(* Logix 5000 Routine export R00_CSV_Control; software revision 36.00 *)

VAR_GLOBAL   (* controller tags *)
   Create_New_CSV_File : BOOL;
   Create_New_CSV_Folder : BOOL;
   CSV_Capture_Rate_Seconds : REAL := 2.0;
   CSV_Data_Logging : BOOL := 1;
   CSV_File_Delay : TIMER := (PRE := 4000);
   CSV_Line_Count_Aux : DINT := 24844;
   CSV_Line_Count_Check_Timer : TIMER := (PRE := 5000);
   CSV_Trigger_2_Pulse : TIMER := (PRE := 1000);
   CSV_Trigger_3_Pulse : TIMER := (PRE := 1000);
   CSV_Update_Pulse : BOOL;
   CSV_Watchdog_Check_Timer : TIMER := (PRE := 5000);
   CurrentWallClock : DINT[7] := ([0] := 2025, [1] := 1, [2] := 19, [3] := 13, [4] := 49, [5] := 30, [6] := 638639);
   Data_Logger_Running : BOOL := 1;
   First_Day_Of_Calendar_Month : BOOL;
   Heartbeat_Off_Time : TIMER := (PRE := 1000);
   Heartbeat_On_Time : TIMER := (PRE := 1000);
   Line_Count : DINT := 50;
   Off_Time : TIMER := (PRE := 5000);
   On_Time : TIMER := (PRE := 100);
   ons_11 : BOOL;
   ONS_4 : BOOL;
   ONS_5 : BOOL;
   ONS_6 : BOOL;
   ONS_7 : BOOL;
   ONS_8 : BOOL := 1;
   ONS_9 : BOOL;
   Pulse_off_Time : TIMER := (PRE := 1700);
   Pulse_On_Time : TIMER := (PRE := 300);
   pulse_time_max : DINT := 3363482;
   SINKRO_File_Name : STRING := 'Report 005 Data';
   SINKRO_Folder_Name : STRING := 'Folder 003';
   SINKRO_Heartbeat : BOOL;
   SINKRO_Line_Count : DINT := 24845;
   SINKRO_New_File : BOOL;
   SINKRO_New_Folder : BOOL;
   SINKRO_Read : BOOL;
   SINKRO_Watchdog : DINT := 92;
   Start_Of_Each_Day : BOOL;
   Temp_Off : BOOL;
   Temp_Off_Time : TIMER := (PRE := 1900);
   Temp_On_Time : TIMER := (PRE := 100);
   Timer_Off_Preset_Aux : DINT := 2000;
   Trigger_1_Temp_Off : BOOL;
   Trigger_1_Timeout : TIMER := (PRE := 2000);
   Watchdog : DINT := 99;
   Watchdog_Check_Pulse : BOOL;
   Watchdog_Max : DINT := 99;
END_VAR

PROGRAM MainProgram
VAR
   CSV_Watchdog_AUx : DINT := 90;
END_VAR

ROUTINE R00_CSV_Control   (* ladder *)
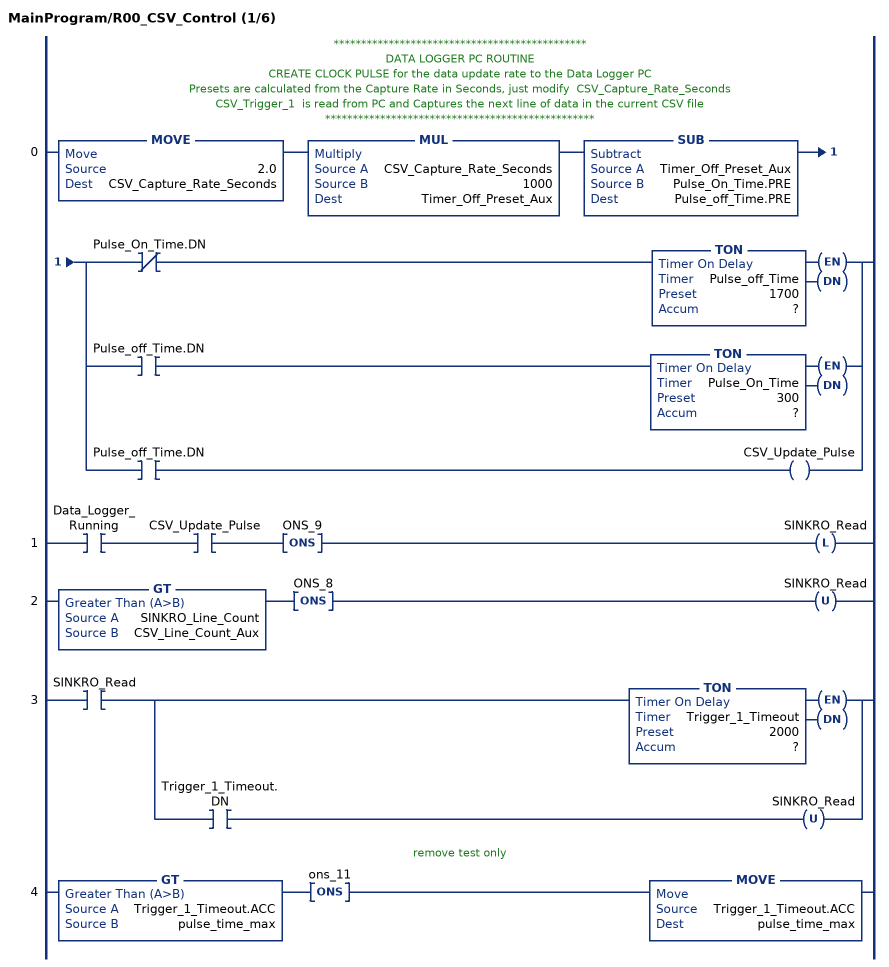
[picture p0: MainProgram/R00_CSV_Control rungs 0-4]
   // **********************************************
   // DATA LOGGER PC ROUTINE
   // CREATE CLOCK PULSE for the data update rate to the Data Logger PC
   // Presets are calculated from the Capture Rate in Seconds, just modify  CSV_Capture_Rate_Seconds
   // CSV_Trigger_1  is read from PC and Captures the next line of data in the current CSV file
   // *************************************************
   0: MOVE(2.0,CSV_Capture_Rate_Seconds)MUL(CSV_Capture_Rate_Seconds,1000,Timer_Off_Preset_Aux)SUB(Timer_Off_Preset_Aux,Pulse_On_Time.PRE,Pulse_off_Time.PRE)[XIO(Pulse_On_Time.DN) TON(Pulse_off_Time,?,?) ,XIC(Pulse_off_Time.DN) TON(Pulse_On_Time,?,?) ,XIC(Pulse_off_Time.DN) OTE(CSV_Update_Pulse) ];
   1: XIC(Data_Logger_Running)XIC(CSV_Update_Pulse)ONS(ONS_9)OTL(SINKRO_Read);
   2: GT(SINKRO_Line_Count,CSV_Line_Count_Aux)ONS(ONS_8)OTU(SINKRO_Read);
   3: XIC(SINKRO_Read)[TON(Trigger_1_Timeout,?,?) ,XIC(Trigger_1_Timeout.DN) OTU(SINKRO_Read) ];
   // remove test only
   4: GT(Trigger_1_Timeout.ACC,pulse_time_max)ONS(ons_11)MOVE(Trigger_1_Timeout.ACC,pulse_time_max);
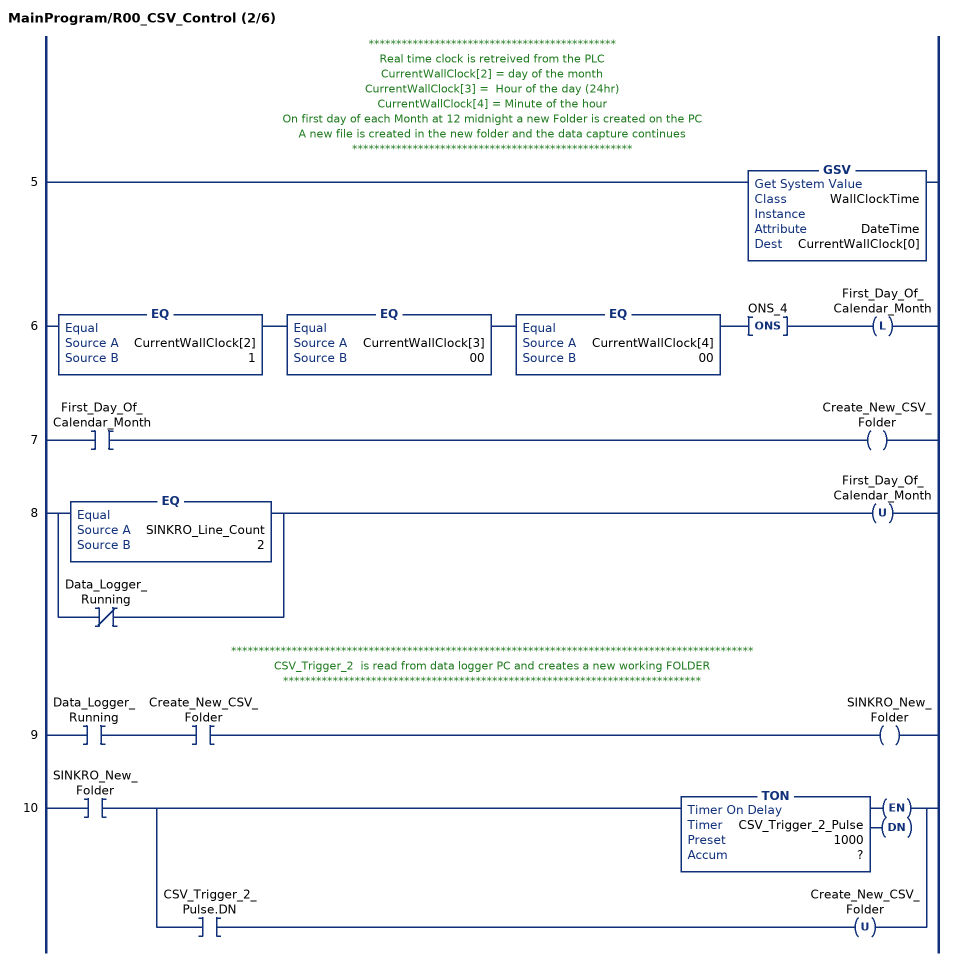
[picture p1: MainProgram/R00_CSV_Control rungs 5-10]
   // *********************************************
   // Real time clock is retreived from the PLC
   // CurrentWallClock[2] = day of the month
   //           CurrentWallClock[3] =  Hour of the day (24hr)
   //   CurrentWallClock[4] = Minute of the hour
   // On first day of each Month at 12 midnight a new Folder is created on the PC
   // A new file is created in the new folder and the data capture continues
   // ***************************************************
   5: GSV(WallClockTime,,DateTime,CurrentWallClock[0]);
   6: EQ(CurrentWallClock[2],1)EQ(CurrentWallClock[3],00)EQ(CurrentWallClock[4],00)ONS(ONS_4)OTL(First_Day_Of_Calendar_Month);
   7: XIC(First_Day_Of_Calendar_Month)OTE(Create_New_CSV_Folder);
   8: [EQ(SINKRO_Line_Count,2) ,XIO(Data_Logger_Running) ]OTU(First_Day_Of_Calendar_Month);
   // ***********************************************************************************************
   // CSV_Trigger_2  is read from data logger PC and creates a new working FOLDER
   // ****************************************************************************
   9: XIC(Data_Logger_Running)XIC(Create_New_CSV_Folder)OTE(SINKRO_New_Folder);
   10: XIC(SINKRO_New_Folder)[TON(CSV_Trigger_2_Pulse,?,?) ,XIC(CSV_Trigger_2_Pulse.DN) OTU(Create_New_CSV_Folder) ];
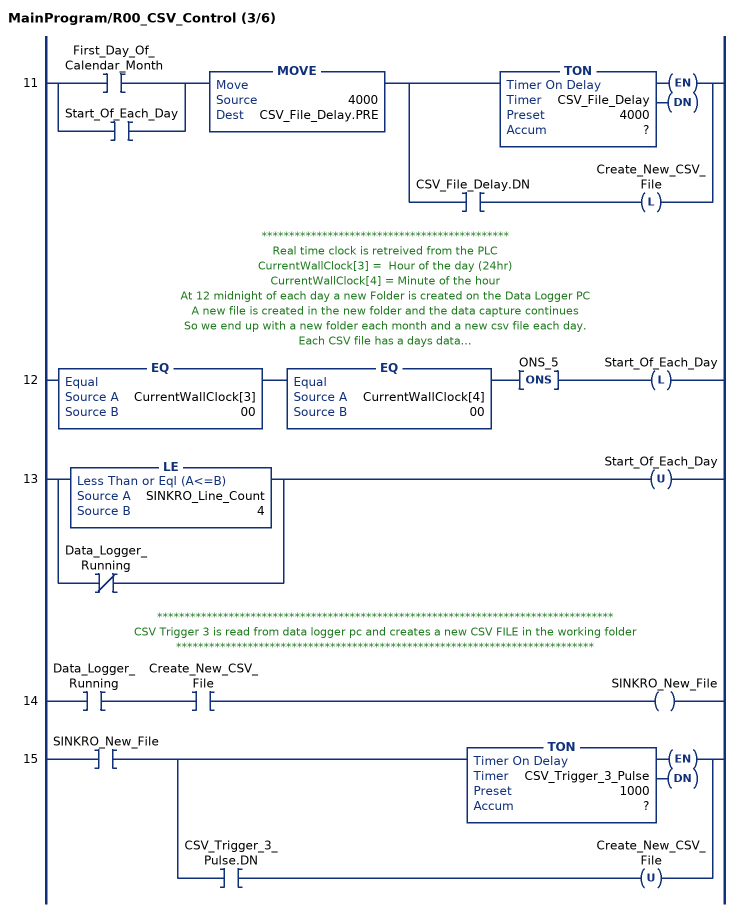
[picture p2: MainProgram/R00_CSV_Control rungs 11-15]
   11: [XIC(First_Day_Of_Calendar_Month) ,XIC(Start_Of_Each_Day) ]MOVE(4000,CSV_File_Delay.PRE)[TON(CSV_File_Delay,?,?) ,XIC(CSV_File_Delay.DN) OTL(Create_New_CSV_File) ];
   // *********************************************
   // Real time clock is retreived from the PLC
   //           CurrentWallClock[3] =  Hour of the day (24hr)
   //   CurrentWallClock[4] = Minute of the hour
   // At 12 midnight of each day a new Folder is created on the Data Logger PC
   // A new file is created in the new folder and the data capture continues
   // So we end up with a new folder each month and a new csv file each day.
   // Each CSV file has a days data.
   // ***************************************************
   12: EQ(CurrentWallClock[3],00)EQ(CurrentWallClock[4],00)ONS(ONS_5)OTL(Start_Of_Each_Day);
   13: [LE(SINKRO_Line_Count,4) ,XIO(Data_Logger_Running) ]OTU(Start_Of_Each_Day);
   // ***********************************************************************************
   // CSV Trigger 3 is read from data logger pc and creates a new CSV FILE in the working folder
   // ****************************************************************************
   14: XIC(Data_Logger_Running)XIC(Create_New_CSV_File)OTE(SINKRO_New_File);
   15: XIC(SINKRO_New_File)[TON(CSV_Trigger_3_Pulse,?,?) ,XIC(CSV_Trigger_3_Pulse.DN) OTU(Create_New_CSV_File) ];
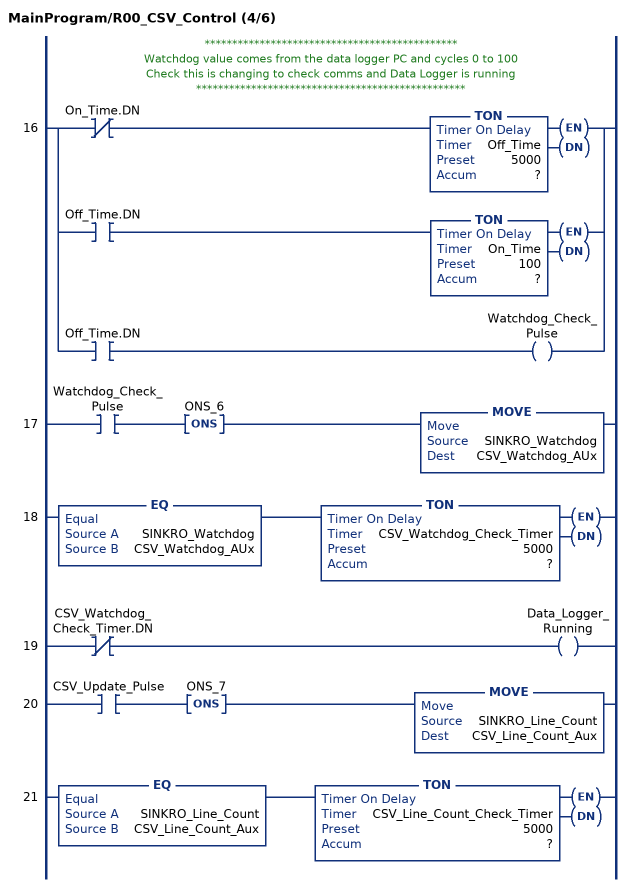
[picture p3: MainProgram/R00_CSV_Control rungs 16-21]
   // **********************************************
   // Watchdog value comes from the data logger PC and cycles 0 to 100
   // Check this is changing to check comms and Data Logger is running
   // *************************************************
   16: [XIO(On_Time.DN) TON(Off_Time,?,?) ,XIC(Off_Time.DN) TON(On_Time,?,?) ,XIC(Off_Time.DN) OTE(Watchdog_Check_Pulse) ];
   17: XIC(Watchdog_Check_Pulse)ONS(ONS_6)MOVE(SINKRO_Watchdog,CSV_Watchdog_AUx);
   18: EQ(SINKRO_Watchdog,CSV_Watchdog_AUx)TON(CSV_Watchdog_Check_Timer,?,?);
   19: XIO(CSV_Watchdog_Check_Timer.DN)OTE(Data_Logger_Running);
   20: XIC(CSV_Update_Pulse)ONS(ONS_7)MOVE(SINKRO_Line_Count,CSV_Line_Count_Aux);
   21: EQ(SINKRO_Line_Count,CSV_Line_Count_Aux)TON(CSV_Line_Count_Check_Timer,?,?);
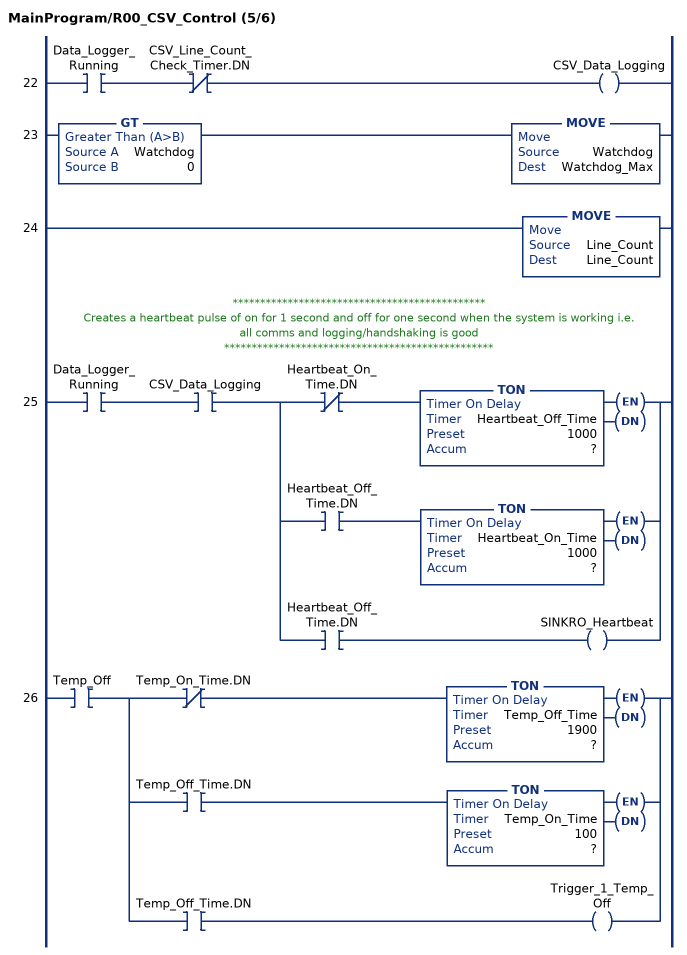
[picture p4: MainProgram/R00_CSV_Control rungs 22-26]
   22: XIC(Data_Logger_Running)XIO(CSV_Line_Count_Check_Timer.DN)OTE(CSV_Data_Logging);
   23: GT(Watchdog,0)MOVE(Watchdog,Watchdog_Max);
   24: MOVE(Line_Count,Line_Count);
   // **********************************************
   // Creates a heartbeat pulse of on for 1 second and off for one second when the system is working i.e.  all comms and logging/handshaking is good
   // *************************************************
   25: XIC(Data_Logger_Running)XIC(CSV_Data_Logging)[XIO(Heartbeat_On_Time.DN) TON(Heartbeat_Off_Time,?,?) ,XIC(Heartbeat_Off_Time.DN) TON(Heartbeat_On_Time,?,?) ,XIC(Heartbeat_Off_Time.DN) OTE(SINKRO_Heartbeat) ];
   26: XIC(Temp_Off)[XIO(Temp_On_Time.DN) TON(Temp_Off_Time,?,?) ,XIC(Temp_Off_Time.DN) TON(Temp_On_Time,?,?) ,XIC(Temp_Off_Time.DN) OTE(Trigger_1_Temp_Off) ];
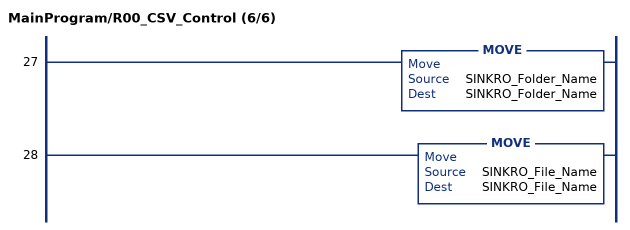
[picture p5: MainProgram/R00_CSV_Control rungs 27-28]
   27: MOVE(SINKRO_Folder_Name,SINKRO_Folder_Name);
   28: MOVE(SINKRO_File_Name,SINKRO_File_Name);
END_ROUTINE
END_PROGRAM
